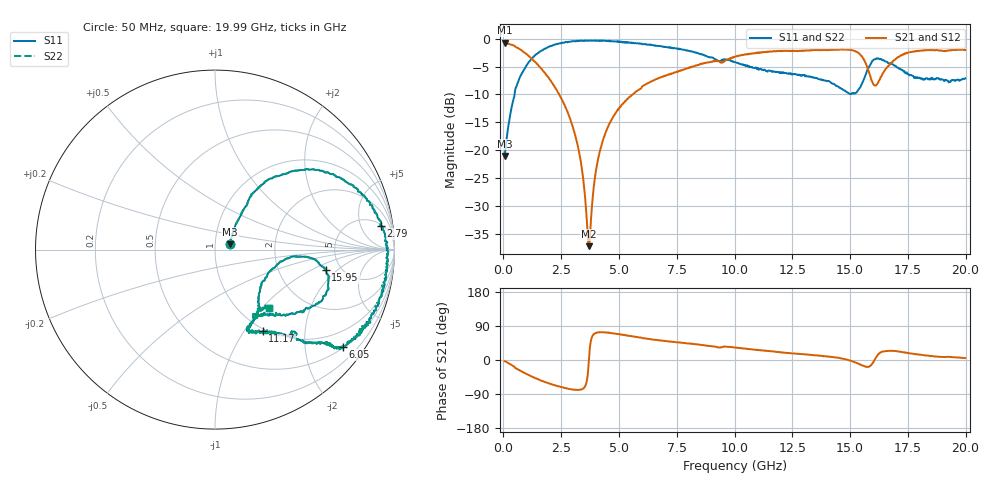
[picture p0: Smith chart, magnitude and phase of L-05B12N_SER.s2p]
! Data Taken on a HP 8720C VNA using a series-through fixture with TRL* de-embedding
#	mhz	s	ma	r	50
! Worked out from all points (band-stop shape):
!   998 points, 50 MHz to 19.99 GHz, reference 50 ohm
!   highest |S21| = -0.70 dB at 50 MHz (marker M1); lowest = -37.2 dB at 3.69 GHz (marker M2)
!   |S21| within 3 dB of the highest: 9.71 GHz to 15.59 GHz (5.884 GHz wide, 46.5 % of centre); 16.95 GHz to end of sweep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
!   lowest |S11| = -21.0 dB at 50 MHz (marker M3), VSWR 1.20, Z = 59 + j3.59 ohm
!   |S11| at or under -10 dB: start of sweep to 480.3 MHz
!   |S22| runs from -21.0 to -0.3 dB; largest |S21 - S12| = 0
!   S11 on the Smith chart (normalised r, x): 50 MHz: 1.18, +0.07; 2.79 GHz: 6, +12; 6.05 GHz: 0.53, -2.87; 11.17 GHz: 0.97, -1.22; 15.95 GHz: 3.81, -1.42; 19.99 GHz: 1.35, -1.09
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50  0.08893 19.8  0.9225 -3.1  0.9225 -3.1  0.08893 19.8
470  0.304 54.4  0.8663 -17.6  0.8663 -17.6  0.304 54.4
830  0.5028 52.0  0.7746 -31.4  0.7746 -31.4  0.5028 52.0
1570  0.7654 33.8  0.5598 -52.9  0.5598 -52.9  0.7654 33.8
2790  0.9344 8.1  0.216 -75.5  0.216 -75.5  0.9344 8.1
3390  0.9584 -1.6  0.06883 -77.4  0.06883 -77.4  0.9584 -1.6
3690  0.96 -5.6  0.01374 -7.0  0.01374 -7.0  0.96 -5.6
4010  0.9642 -10.4  0.06683 71.7  0.06683 71.7  0.9642 -10.4
4390  0.9574 -16.1  0.1384 72.9  0.1384 72.9  0.9574 -16.1
4950  0.9556 -25.1  0.2332 68.7  0.2332 68.7  0.9556 -25.1
6050  0.8942 -37.3  0.3794 57.6  0.3794 57.6  0.8942 -37.3
6710  0.862 -39.1  0.4421 52.4  0.4421 52.4  0.862 -39.1
10030  0.6173 -50.6  0.6925 33.1  0.6925 33.1  0.6173 -50.6
11170  0.5264 -59.8  0.7507 25.4  0.7507 25.4  0.5264 -59.8
13350  0.4506 -62.1  0.7884 12.8  0.7884 12.8  0.4506 -62.1
15130  0.3217 -29.3  0.7861 -4.2  0.7861 -4.2  0.3217 -29.3
15630  0.4499 -4.9  0.6311 -16.9  0.6311 -16.9  0.4499 -4.9
15950  0.6281 -10.4  0.4164 -10.2  0.4164 -10.2  0.6281 -10.4
16310  0.66 -24.2  0.444 20.1  0.444 20.1  0.66 -24.2
16670  0.6019 -32.7  0.5728 24.1  0.5728 24.1  0.6019 -32.7
18210  0.4346 -58.8  0.7899 12.3  0.7899 12.3  0.4346 -58.8
19990  0.442 -47.2  0.7927 5.1  0.7927 5.1  0.442 -47.2
